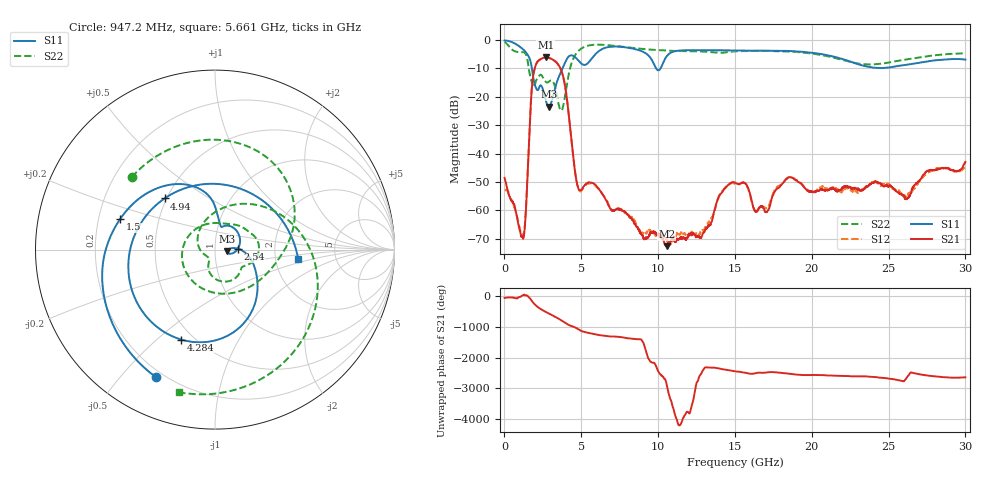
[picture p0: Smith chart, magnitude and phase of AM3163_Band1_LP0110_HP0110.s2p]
!Agilent Technologies,E8364B,MY43040894,A.07.50.67
!Agilent E8364B: A.07.50.67
!Date: Thursday, August 20, 2020 11:17:50
!Correction: S11(Full 2 Port(1,2))
!S21(Full 2 Port(1,2))
!S12(Full 2 Port(1,2))
!S22(Full 2 Port(1,2))
!S2P File: Measurements: S11, S21, S12, S22:
# Hz S  dB  R 50
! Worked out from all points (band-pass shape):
!   3201 points, 10 MHz to 30 GHz, reference 50 ohm
!   highest |S21| = -6.13 dB at 2.69 GHz (marker M1); lowest = -72.6 dB at 10.56 GHz (marker M2)
!   |S21| within 3 dB of the highest: 2.016 GHz to 3.563 GHz (1.547 GHz wide, 55.5 % of centre)
!   lowest |S11| = -23.5 dB at 2.897 GHz (marker M3), VSWR 1.14, Z = 57.1 - j1.1 ohm
!   |S11| at or under -10 dB: 1.786 GHz to 3.778 GHz (1.992 GHz wide, 71.6 % of centre); 9.874 GHz to 10.16 GHz (282.9 MHz wide, 2.82 % of centre)
!   |S22| runs from -24.9 to -0.6 dB; largest |S21 - S12| = 0.0035
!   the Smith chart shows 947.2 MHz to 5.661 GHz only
!   S11 on the Smith chart (normalised r, x): 947.2 MHz: 0.17, -0.63; 1.5 GHz: 0.29, +0.14; 2.54 GHz: 1.29, +0.00; 4.284 GHz: 0.43, -0.60; 4.94 GHz: 0.49, +0.33; 5.661 GHz: 2.69, -0.38
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1e7  -0.12 -7.8  -48.57 -49.2  -52.99 14.0  -0.61 -23.8
5.160812e8  -0.76 -61.8  -56.73 -38.7  -57.41 -42.4  -3.42 -143.6
9.471875e8  -2.12 -114.8  -65.94 -22.9  -65.06 49.5  -4.22 138.9
1.500128e9  -5.10 162.3  -48.57 21.7  -47.87 25.8  -7.00 14.1
1.884375e9  -13.53 87.5  -12.16 145.2  -12.16 145.2  -16.48 110.1
2.540406e9  -18.03 0.8  -6.25 -107.3  -6.26 -107.4  -13.54 -21.5
2.690356e9  -21.25 -15.4  -6.13 -148.9  -6.13 -148.9  -14.73 -30.3
2.896538e9  -23.48 -8.3  -6.28 156.8  -6.30 156.7  -14.64 -40.3
3.702519e9  -10.92 -34.5  -10.74 -64.0  -10.77 -63.9  -24.86 -133.6
4.283575e9  -5.43 -110.5  -31.32 123.2  -31.28 123.6  -9.63 49.8
4.939606e9  -7.95 134.6  -53.01 -34.1  -53.32 -33.2  -3.20 -43.4
5.014581e9  -8.32 119.5  -52.67 -52.1  -53.10 -51.9  -2.92 -51.0
5.661241e9  -6.61 -6.7  -50.26 -135.6  -50.46 -135.9  -1.72 -104.1
6.448478e9  -2.94 -97.6  -54.82 151.7  -54.83 152.8  -1.66 -151.9
7.488756e9  -2.32 -170.0  -59.78 114.9  -59.50 112.0  -2.21 158.5
1.000979e10  -10.65 89.6  -68.24 61.2  -68.73 97.9  -3.54 60.0
1.056273e10  -5.67 93.2  -72.62 -20.6  -70.28 26.8  -3.71 40.2
1.242773e10  -3.55 6.6  -68.91 -121.3  -68.75 -18.6  -3.96 -22.6
1.5005e10  -3.65 -72.1  -50.21 68.6  -50.58 69.3  -3.95 -90.3
2.000958e10  -4.44 163.3  -53.38 -51.2  -53.40 -53.9  -4.72 136.7
2.500479e10  -9.67 -62.2  -51.71 -169.2  -50.60 -174.3  -7.95 -92.2
3e10  -6.86 104.5  -42.95 -128.1  -44.83 -133.0  -4.66 102.4
